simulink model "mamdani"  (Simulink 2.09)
settings: Solver=ode45  StartTime=0.0  StopTime=20  MaxStep=1  RelTol=1e-3  AbsTol=1e-3

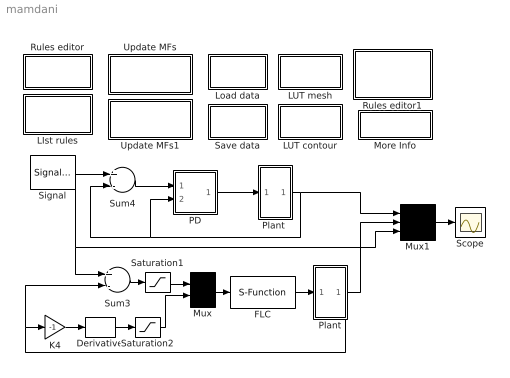
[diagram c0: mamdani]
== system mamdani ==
  " Plant " : Subsystem
  " Plant  " : Subsystem
  Derivative : Derivative
  FLC : S-Function  FunctionName=sfuninf  Parameters=rls, mfs, def  mask(Fuzzy inference block){}
      mask help: MIN-MAX inference with fuzzy means defuzzification
      mask init:
      | rls = @1; mfs = @2; def = @3;
  K4 : Gain  Gain=-1
  LIst rules : Subsystem
  LUT contour : Subsystem
  LUT mesh : Subsystem
  Load data : Subsystem
  More Info : Subsystem
  Mux : Mux  Inputs=2
  Mux1 : Mux  Inputs=3
  PD : Subsystem
      mask help: PID controller
      mask init:
      | P = @1; D = -@2; I = @3;
  Rules editor : Subsystem
  Rules editor1 : Subsystem
  Saturation1 : Saturate  UpperLimit=2  LowerLimit=-2
  Saturation2 : Saturate  UpperLimit=2  LowerLimit=-2
  Save data : Subsystem
  Scope : Scope
  Signal : SignalGenerator  WaveForm=square  Amplitude=1.000000  Frequency=0.500000  Units=rad/sec
  Sum3 : Sum  Inputs=+-
  Sum4 : Sum  Inputs=+-
  Update MFs : Subsystem
  Update MFs1 : Subsystem
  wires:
  Mux1/1 -> Scope/1
  K4/1 -> Derivative/1
  " Plant "/1(out_1) -> Mux1/2, K4/1, Sum3/2
  FLC/1 -> " Plant "/1(in_1)
  PD/1(Out_1) -> " Plant  "/1(in_1)
  Mux/1 -> FLC/1
  Derivative/1 -> Saturation2/1
  Sum3/1 -> Saturation1/1
  Saturation1/1 -> Mux/1
  Saturation2/1 -> Mux/2
  Sum4/1 -> PD/1(In_1)
  " Plant  "/1(out_1) -> Mux1/1, PD/2(In_2), Sum4/2
  Signal/1 -> Mux1/3, Sum3/1, Sum4/1

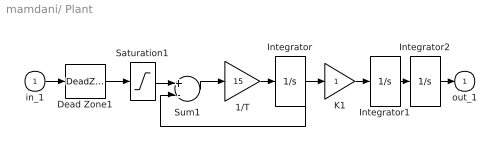
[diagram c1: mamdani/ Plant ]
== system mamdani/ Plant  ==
  in_1 : Inport  Port=1  PortWidth=-1  SampleTime=-1
  1/T : Gain  Gain=15
  Dead Zone1 : DeadZone  LowerValue=-0.1  UpperValue=0.1
  Integrator : Integrator  ExternalReset=none  InitialConditionSource=internal  InitialCondition=0  LimitOutput=off  UpperSaturationLimit=inf  LowerSaturationLimit=-inf  ShowSaturationPort=off  ShowStatePort=off  AbsoluteTolerance=auto
  Integrator1 : Integrator  ExternalReset=none  InitialConditionSource=internal  InitialCondition=0  LimitOutput=off  UpperSaturationLimit=inf  LowerSaturationLimit=-inf  ShowSaturationPort=off  ShowStatePort=off  AbsoluteTolerance=auto
  Integrator2 : Integrator  ExternalReset=none  InitialConditionSource=internal  InitialCondition=0  LimitOutput=off  UpperSaturationLimit=inf  LowerSaturationLimit=-inf  ShowSaturationPort=off  ShowStatePort=off  AbsoluteTolerance=auto
  K1 : Gain  Gain=1
  Saturation1 : Saturate  UpperLimit=1  LowerLimit=-1
  Sum1 : Sum  Inputs=+-
  out_1 : Outport  Port=1  InitialOutput=0
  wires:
  Sum1/1 -> 1/T/1
  1/T/1 -> Integrator/1
  Integrator1/1 -> Integrator2/1
  Integrator/1 -> Sum1/2, K1/1
  K1/1 -> Integrator1/1
  Integrator2/1 -> out_1/1
  in_1/1 -> Dead Zone1/1
  Dead Zone1/1 -> Saturation1/1
  Saturation1/1 -> Sum1/1

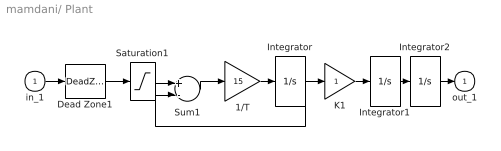
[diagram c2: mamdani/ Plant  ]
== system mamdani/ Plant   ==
  in_1 : Inport  Port=1  PortWidth=-1  SampleTime=-1
  1/T : Gain  Gain=15
  Dead Zone1 : DeadZone  LowerValue=-0.1  UpperValue=0.1
  Integrator : Integrator  ExternalReset=none  InitialConditionSource=internal  InitialCondition=0  LimitOutput=off  UpperSaturationLimit=inf  LowerSaturationLimit=-inf  ShowSaturationPort=off  ShowStatePort=off  AbsoluteTolerance=auto
  Integrator1 : Integrator  ExternalReset=none  InitialConditionSource=internal  InitialCondition=0  LimitOutput=off  UpperSaturationLimit=inf  LowerSaturationLimit=-inf  ShowSaturationPort=off  ShowStatePort=off  AbsoluteTolerance=auto
  Integrator2 : Integrator  ExternalReset=none  InitialConditionSource=internal  InitialCondition=0  LimitOutput=off  UpperSaturationLimit=inf  LowerSaturationLimit=-inf  ShowSaturationPort=off  ShowStatePort=off  AbsoluteTolerance=auto
  K1 : Gain  Gain=1
  Saturation1 : Saturate  UpperLimit=1  LowerLimit=-1
  Sum1 : Sum  Inputs=+-
  out_1 : Outport  Port=1  InitialOutput=0
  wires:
  Saturation1/1 -> Sum1/1
  Dead Zone1/1 -> Saturation1/1
  in_1/1 -> Dead Zone1/1
  Integrator2/1 -> out_1/1
  K1/1 -> Integrator1/1
  Integrator1/1 -> Integrator2/1
  1/T/1 -> Integrator/1
  Sum1/1 -> 1/T/1
  Integrator/1 -> K1/1, Sum1/2

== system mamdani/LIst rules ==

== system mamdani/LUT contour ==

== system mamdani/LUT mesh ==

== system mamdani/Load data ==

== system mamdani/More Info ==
  note: This demonstration compares PD vers. Fuzzy control for a nonlinear third-order plant.
  note: To strart click on "Compile rule-base" first. On other systems than MS-Windows, you may want to change the "Edit rules" icon in order to set your preferred text editor. Experiment with changing membership functions and rules.

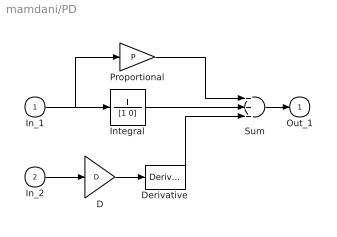
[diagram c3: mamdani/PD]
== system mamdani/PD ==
  In_1 : Inport  Port=1  PortWidth=-1  SampleTime=-1
  In_2 : Inport  Port=2  PortWidth=-1  SampleTime=-1
  D : Gain  Gain=D
  Derivative : Derivative
  Integral : TransferFcn  Numerator=I  Denominator=[1 0]
  Proportional : Gain  Gain=P
  Sum : Sum  Inputs=+++
  Out_1 : Outport  Port=1  InitialOutput=0
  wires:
  In_2/1 -> D/1
  Proportional/1 -> Sum/1
  Integral/1 -> Sum/2
  Derivative/1 -> Sum/3
  In_1/1 -> Integral/1, Proportional/1
  Sum/1 -> Out_1/1
  D/1 -> Derivative/1

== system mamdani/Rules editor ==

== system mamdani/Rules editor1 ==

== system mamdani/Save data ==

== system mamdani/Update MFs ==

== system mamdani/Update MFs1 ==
